(* Logix 5000 AddOnInstructionDefinition export Banner_T30RKU_Param_v4; software revision 33.00; part 2 of 3 *)
(* tags used below, declared in another part *)
   T30RKU : Banner_T30RKU_v4;
   Port_Data : Banner_IOL_Port_v4;
   Port : DINT;
   Local_Control : DINT;
   Command_Being_Processed : BOOL;
   Update_Archive : BOOL;
   Index_Write_Inprocess : DINT;
   Index_Write_Control : DINT;
   Inprocess_Index : DINT;
(* Banner_T30RKU_Param_v4, continued *)

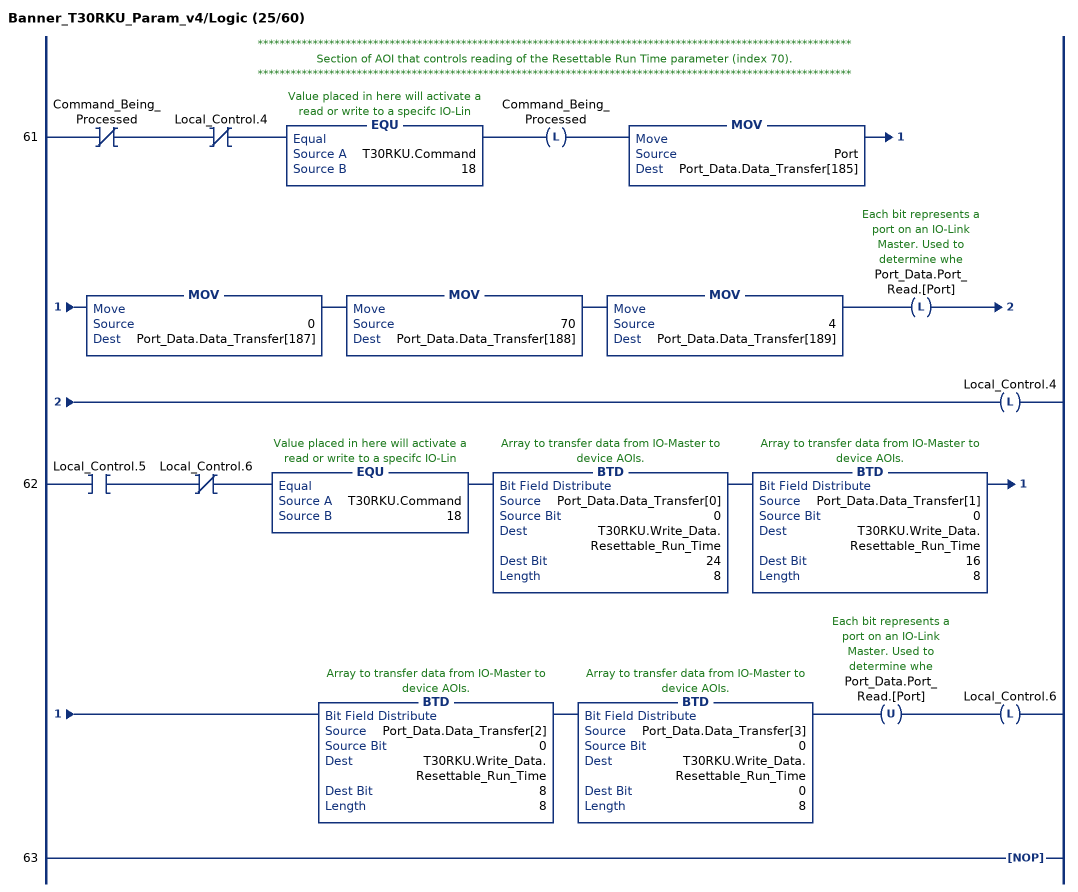
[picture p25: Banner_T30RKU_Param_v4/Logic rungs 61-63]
   // ************************************************************************************************************
   // Section of AOI that controls reading of the Resettable Run Time parameter (index 70).
   // ************************************************************************************************************
   61: XIO(Command_Being_Processed)XIO(Local_Control.4)EQU(T30RKU.Command,18)OTL(Command_Being_Processed)MOV(Port,Port_Data.Data_Transfer[185])MOV(0,Port_Data.Data_Transfer[187])MOV(70,Port_Data.Data_Transfer[188])MOV(4,Port_Data.Data_Transfer[189])OTL(Port_Data.Port_Read.[Port])OTL(Local_Control.4);
   62: XIC(Local_Control.5)XIO(Local_Control.6)EQU(T30RKU.Command,18)BTD(Port_Data.Data_Transfer[0],0,T30RKU.Write_Data.Resettable_Run_Time,24,8)BTD(Port_Data.Data_Transfer[1],0,T30RKU.Write_Data.Resettable_Run_Time,16,8)BTD(Port_Data.Data_Transfer[2],0,T30RKU.Write_Data.Resettable_Run_Time,8,8)BTD(Port_Data.Data_Transfer[3],0,T30RKU.Write_Data.Resettable_Run_Time,0,8)OTU(Port_Data.Port_Read.[Port])OTL(Local_Control.6);
   63: NOP();
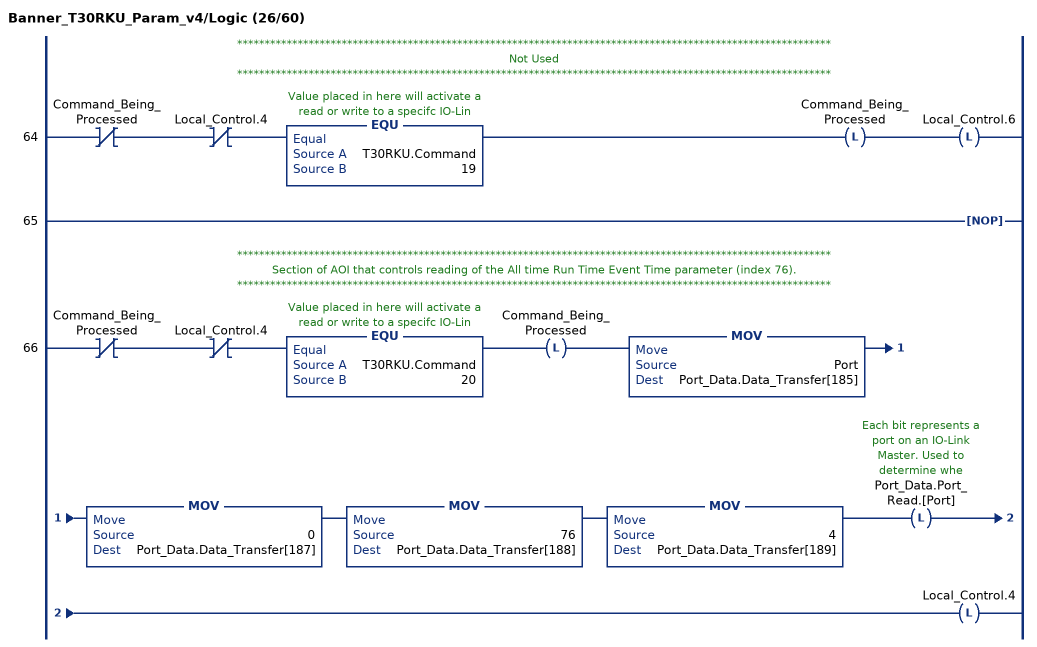
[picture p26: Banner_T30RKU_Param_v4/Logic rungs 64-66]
   // ************************************************************************************************************
   // Not Used
   // ************************************************************************************************************
   64: XIO(Command_Being_Processed)XIO(Local_Control.4)EQU(T30RKU.Command,19)OTL(Command_Being_Processed)OTL(Local_Control.6);
   65: NOP();
   // ************************************************************************************************************
   // Section of AOI that controls reading of the All time Run Time Event Time parameter (index 76).
   // ************************************************************************************************************
   66: XIO(Command_Being_Processed)XIO(Local_Control.4)EQU(T30RKU.Command,20)OTL(Command_Being_Processed)MOV(Port,Port_Data.Data_Transfer[185])MOV(0,Port_Data.Data_Transfer[187])MOV(76,Port_Data.Data_Transfer[188])MOV(4,Port_Data.Data_Transfer[189])OTL(Port_Data.Port_Read.[Port])OTL(Local_Control.4);
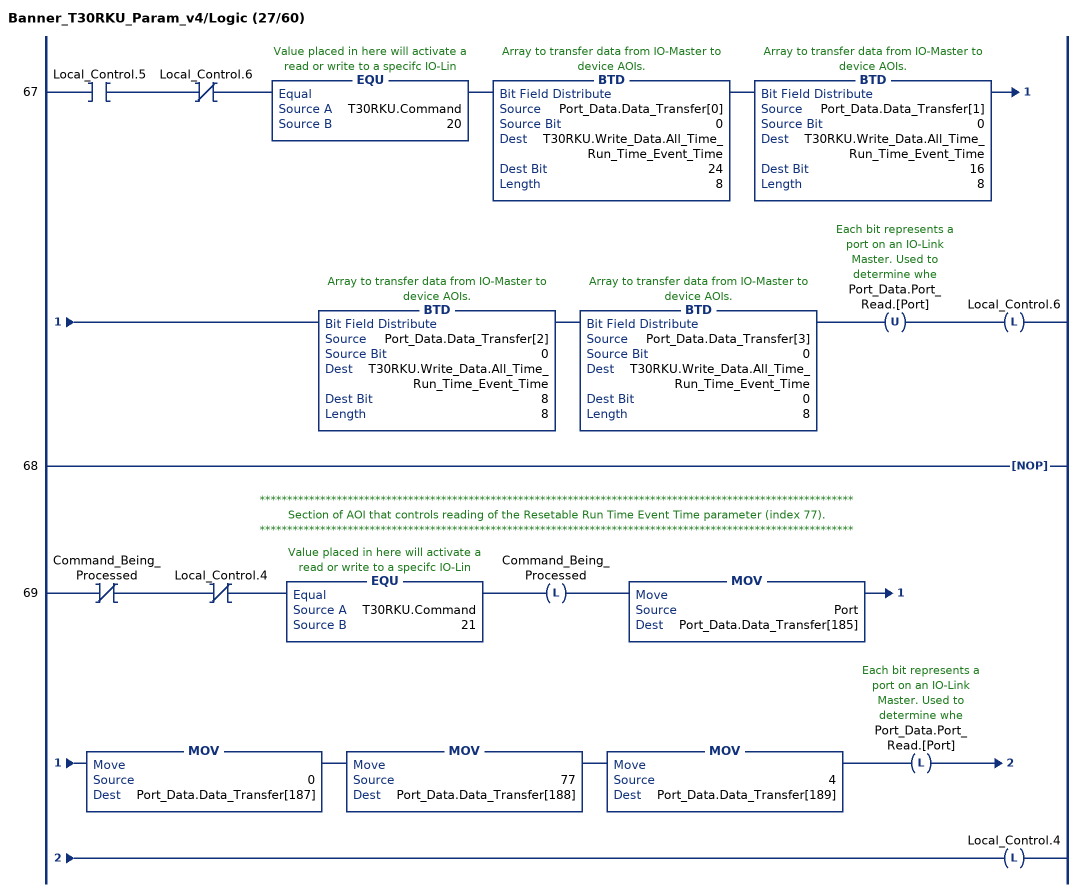
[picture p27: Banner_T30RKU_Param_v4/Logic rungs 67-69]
   67: XIC(Local_Control.5)XIO(Local_Control.6)EQU(T30RKU.Command,20)BTD(Port_Data.Data_Transfer[0],0,T30RKU.Write_Data.All_Time_Run_Time_Event_Time,24,8)BTD(Port_Data.Data_Transfer[1],0,T30RKU.Write_Data.All_Time_Run_Time_Event_Time,16,8)BTD(Port_Data.Data_Transfer[2],0,T30RKU.Write_Data.All_Time_Run_Time_Event_Time,8,8)BTD(Port_Data.Data_Transfer[3],0,T30RKU.Write_Data.All_Time_Run_Time_Event_Time,0,8)OTU(Port_Data.Port_Read.[Port])OTL(Local_Control.6);
   68: NOP();
   // ************************************************************************************************************
   // Section of AOI that controls reading of the Resetable Run Time Event Time parameter (index 77).
   // ************************************************************************************************************
   69: XIO(Command_Being_Processed)XIO(Local_Control.4)EQU(T30RKU.Command,21)OTL(Command_Being_Processed)MOV(Port,Port_Data.Data_Transfer[185])MOV(0,Port_Data.Data_Transfer[187])MOV(77,Port_Data.Data_Transfer[188])MOV(4,Port_Data.Data_Transfer[189])OTL(Port_Data.Port_Read.[Port])OTL(Local_Control.4);
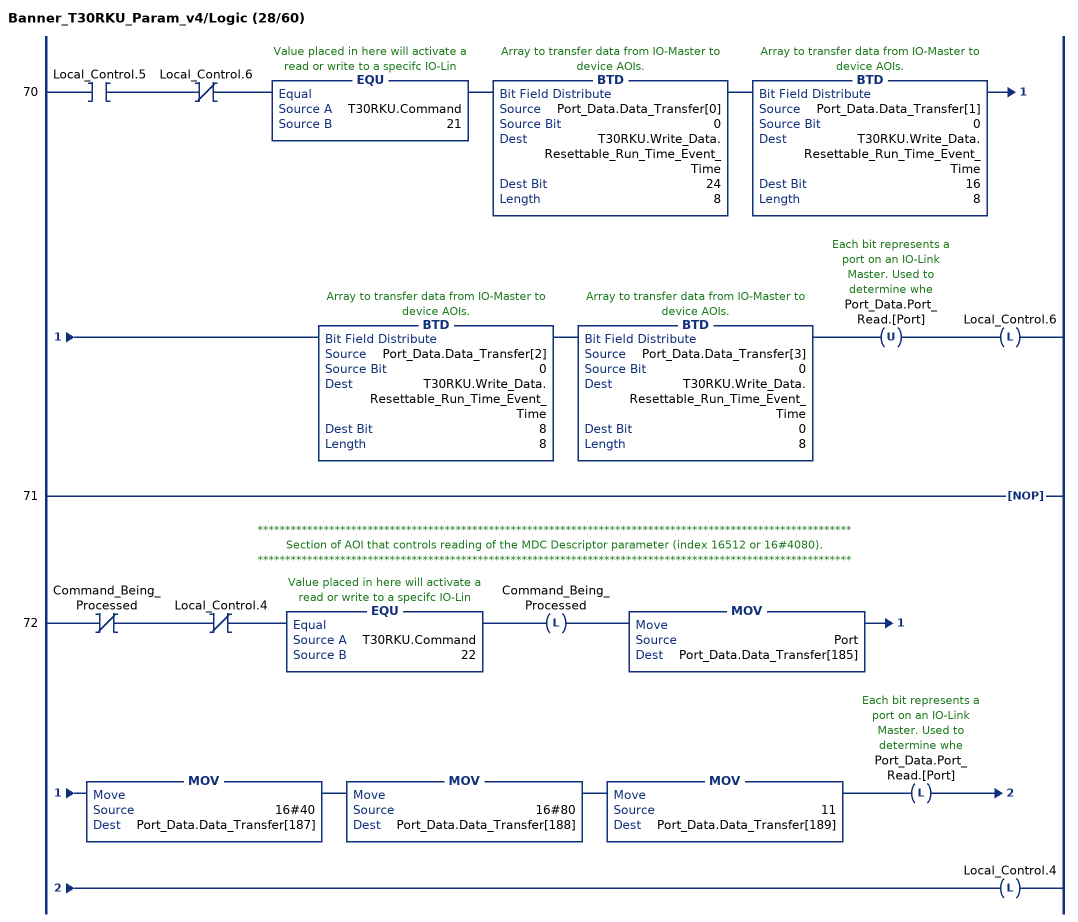
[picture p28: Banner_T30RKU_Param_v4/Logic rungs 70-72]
   70: XIC(Local_Control.5)XIO(Local_Control.6)EQU(T30RKU.Command,21)BTD(Port_Data.Data_Transfer[0],0,T30RKU.Write_Data.Resettable_Run_Time_Event_Time,24,8)BTD(Port_Data.Data_Transfer[1],0,T30RKU.Write_Data.Resettable_Run_Time_Event_Time,16,8)BTD(Port_Data.Data_Transfer[2],0,T30RKU.Write_Data.Resettable_Run_Time_Event_Time,8,8)BTD(Port_Data.Data_Transfer[3],0,T30RKU.Write_Data.Resettable_Run_Time_Event_Time,0,8)OTU(Port_Data.Port_Read.[Port])OTL(Local_Control.6);
   71: NOP();
   // ************************************************************************************************************
   // Section of AOI that controls reading of the MDC Descriptor parameter (index 16512 or 16#4080).
   // ************************************************************************************************************
   72: XIO(Command_Being_Processed)XIO(Local_Control.4)EQU(T30RKU.Command,22)OTL(Command_Being_Processed)MOV(Port,Port_Data.Data_Transfer[185])MOV(16#40,Port_Data.Data_Transfer[187])MOV(16#80,Port_Data.Data_Transfer[188])MOV(11,Port_Data.Data_Transfer[189])OTL(Port_Data.Port_Read.[Port])OTL(Local_Control.4);
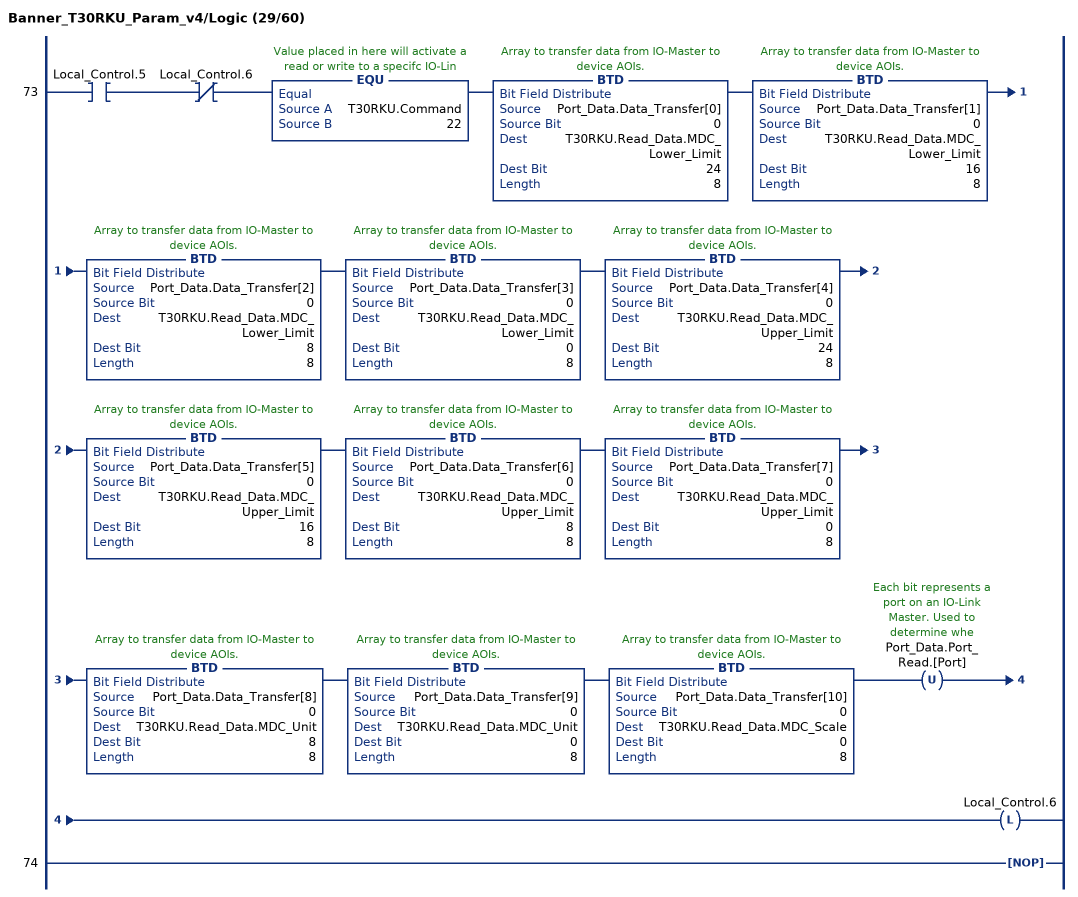
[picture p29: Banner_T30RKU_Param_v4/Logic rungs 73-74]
   73: XIC(Local_Control.5)XIO(Local_Control.6)EQU(T30RKU.Command,22)BTD(Port_Data.Data_Transfer[0],0,T30RKU.Read_Data.MDC_Lower_Limit,24,8)BTD(Port_Data.Data_Transfer[1],0,T30RKU.Read_Data.MDC_Lower_Limit,16,8)BTD(Port_Data.Data_Transfer[2],0,T30RKU.Read_Data.MDC_Lower_Limit,8,8)BTD(Port_Data.Data_Transfer[3],0,T30RKU.Read_Data.MDC_Lower_Limit,0,8)BTD(Port_Data.Data_Transfer[4],0,T30RKU.Read_Data.MDC_Upper_Limit,24,8)BTD(Port_Data.Data_Transfer[5],0,T30RKU.Read_Data.MDC_Upper_Limit,16,8)BTD(Port_Data.Data_Transfer[6],0,T30RKU.Read_Data.MDC_Upper_Limit,8,8)BTD(Port_Data.Data_Transfer[7],0,T30RKU.Read_Data.MDC_Upper_Limit,0,8)BTD(Port_Data.Data_Transfer[8],0,T30RKU.Read_Data.MDC_Unit,8,8)BTD(Port_Data.Data_Transfer[9],0,T30RKU.Read_Data.MDC_Unit,0,8)BTD(Port_Data.Data_Transfer[10],0,T30RKU.Read_Data.MDC_Scale,0,8)OTU(Port_Data.Port_Read.[Port])OTL(Local_Control.6);
   74: NOP();
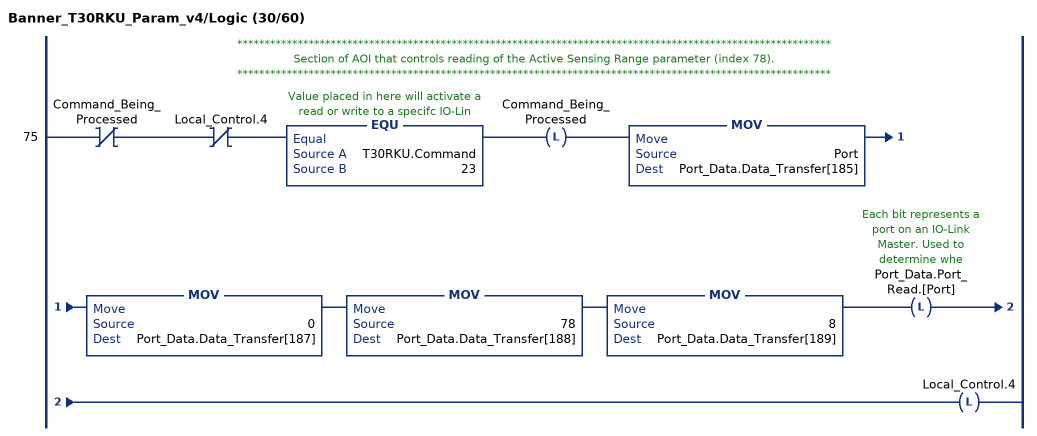
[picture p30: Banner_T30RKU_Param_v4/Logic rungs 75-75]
   // ************************************************************************************************************
   // Section of AOI that controls reading of the Active Sensing Range parameter (index 78).
   // ************************************************************************************************************
   75: XIO(Command_Being_Processed)XIO(Local_Control.4)EQU(T30RKU.Command,23)OTL(Command_Being_Processed)MOV(Port,Port_Data.Data_Transfer[185])MOV(0,Port_Data.Data_Transfer[187])MOV(78,Port_Data.Data_Transfer[188])MOV(8,Port_Data.Data_Transfer[189])OTL(Port_Data.Port_Read.[Port])OTL(Local_Control.4);
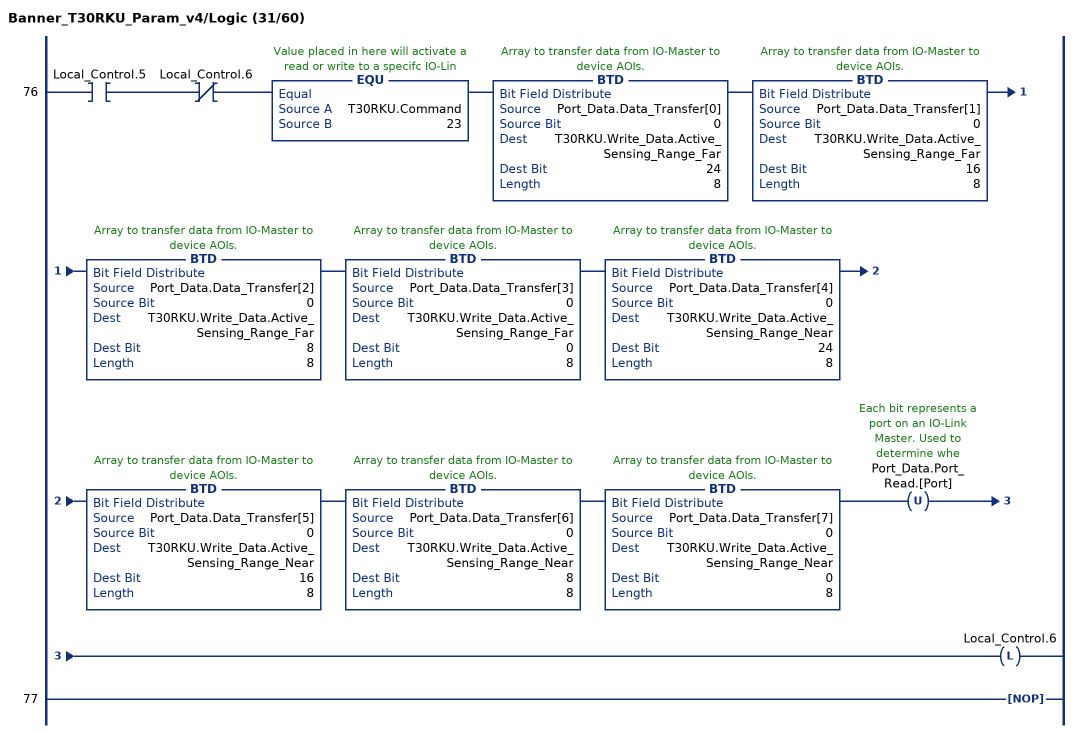
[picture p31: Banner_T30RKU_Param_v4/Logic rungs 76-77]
   76: XIC(Local_Control.5)XIO(Local_Control.6)EQU(T30RKU.Command,23)BTD(Port_Data.Data_Transfer[0],0,T30RKU.Write_Data.Active_Sensing_Range_Far,24,8)BTD(Port_Data.Data_Transfer[1],0,T30RKU.Write_Data.Active_Sensing_Range_Far,16,8)BTD(Port_Data.Data_Transfer[2],0,T30RKU.Write_Data.Active_Sensing_Range_Far,8,8)BTD(Port_Data.Data_Transfer[3],0,T30RKU.Write_Data.Active_Sensing_Range_Far,0,8)BTD(Port_Data.Data_Transfer[4],0,T30RKU.Write_Data.Active_Sensing_Range_Near,24,8)BTD(Port_Data.Data_Transfer[5],0,T30RKU.Write_Data.Active_Sensing_Range_Near,16,8)BTD(Port_Data.Data_Transfer[6],0,T30RKU.Write_Data.Active_Sensing_Range_Near,8,8)BTD(Port_Data.Data_Transfer[7],0,T30RKU.Write_Data.Active_Sensing_Range_Near,0,8)OTU(Port_Data.Port_Read.[Port])OTL(Local_Control.6);
   77: NOP();
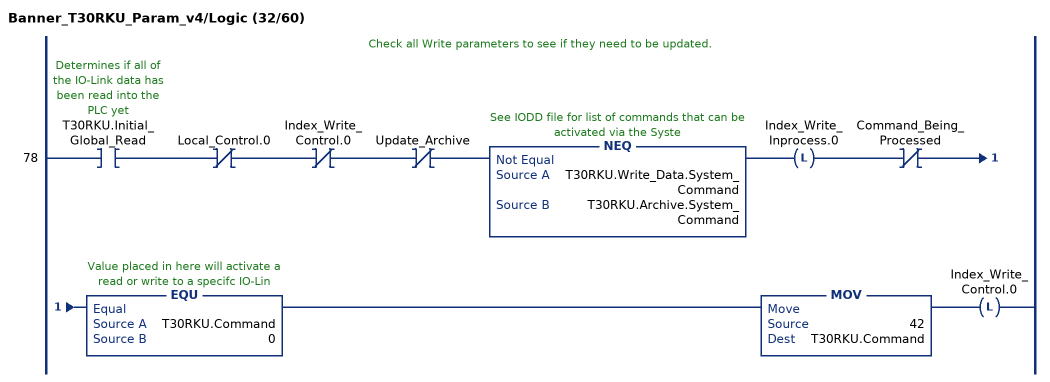
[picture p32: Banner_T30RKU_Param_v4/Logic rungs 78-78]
   // Check all Write parameters to see if they need to be updated.
   78: XIC(T30RKU.Initial_Global_Read)XIO(Local_Control.0)XIO(Index_Write_Control.0)XIO(Update_Archive)NEQ(T30RKU.Write_Data.System_Command,T30RKU.Archive.System_Command)OTL(Index_Write_Inprocess.0)XIO(Command_Being_Processed)EQU(T30RKU.Command,0)MOV(42,T30RKU.Command)OTL(Index_Write_Control.0);
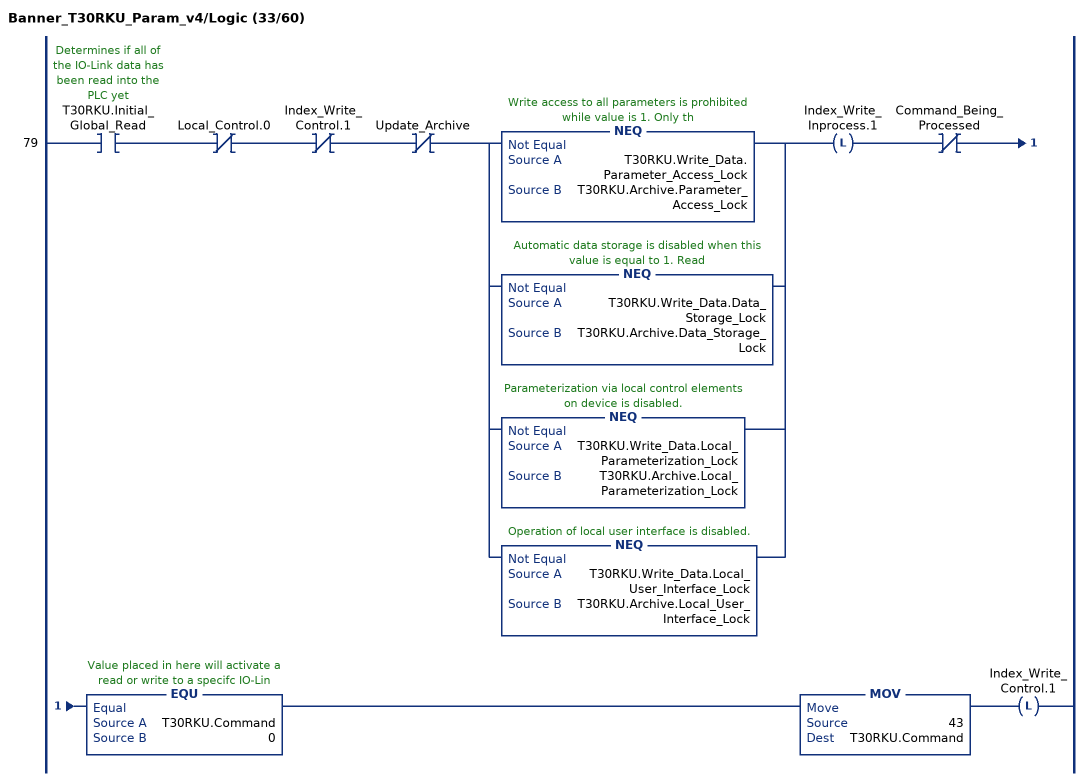
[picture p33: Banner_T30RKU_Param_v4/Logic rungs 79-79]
   79: XIC(T30RKU.Initial_Global_Read)XIO(Local_Control.0)XIO(Index_Write_Control.1)XIO(Update_Archive)[NEQ(T30RKU.Write_Data.Parameter_Access_Lock,T30RKU.Archive.Parameter_Access_Lock) ,NEQ(T30RKU.Write_Data.Data_Storage_Lock,T30RKU.Archive.Data_Storage_Lock) ,NEQ(T30RKU.Write_Data.Local_Parameterization_Lock,T30RKU.Archive.Local_Parameterization_Lock) ,NEQ(T30RKU.Write_Data.Local_User_Interface_Lock,T30RKU.Archive.Local_User_Interface_Lock) ]OTL(Index_Write_Inprocess.1)XIO(Command_Being_Processed)EQU(T30RKU.Command,0)MOV(43,T30RKU.Command)OTL(Index_Write_Control.1);
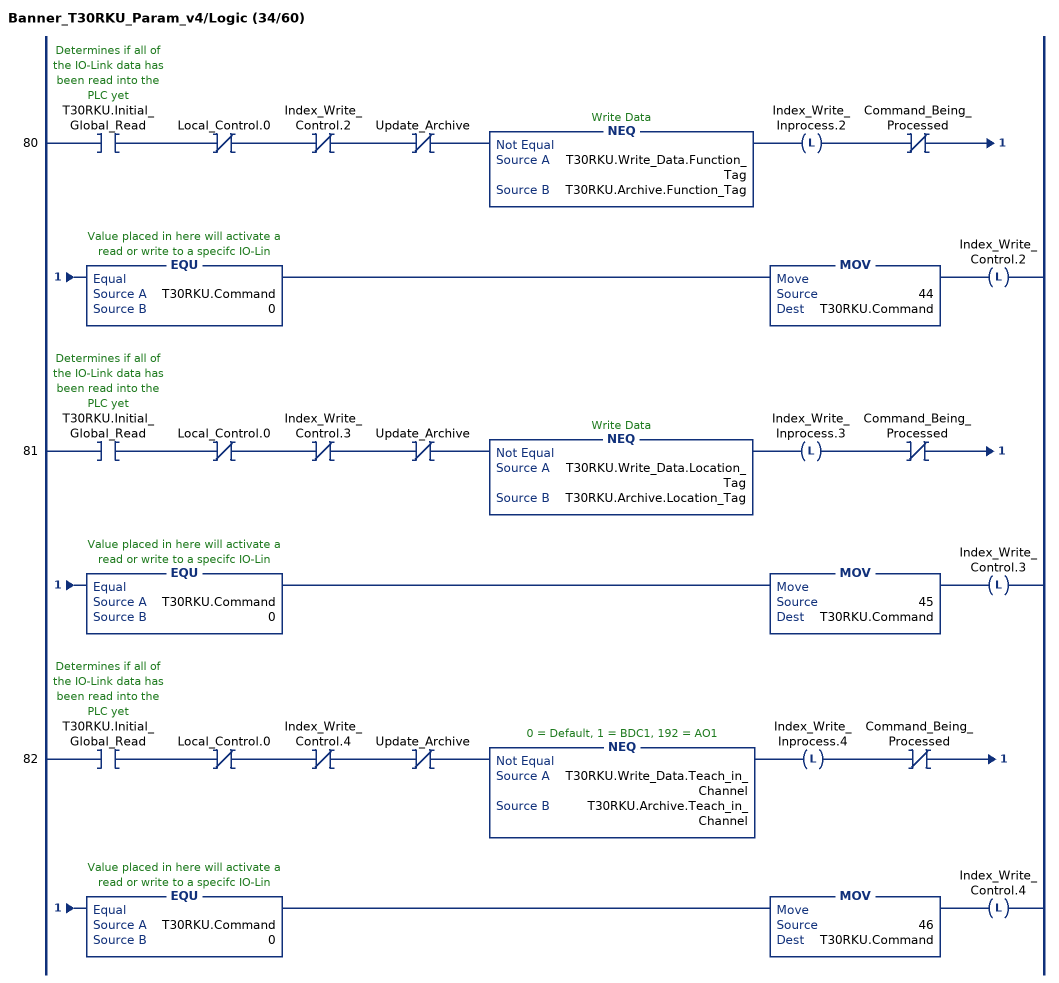
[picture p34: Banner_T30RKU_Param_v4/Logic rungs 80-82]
   80: XIC(T30RKU.Initial_Global_Read)XIO(Local_Control.0)XIO(Index_Write_Control.2)XIO(Update_Archive)NEQ(T30RKU.Write_Data.Function_Tag,T30RKU.Archive.Function_Tag)OTL(Index_Write_Inprocess.2)XIO(Command_Being_Processed)EQU(T30RKU.Command,0)MOV(44,T30RKU.Command)OTL(Index_Write_Control.2);
   81: XIC(T30RKU.Initial_Global_Read)XIO(Local_Control.0)XIO(Index_Write_Control.3)XIO(Update_Archive)NEQ(T30RKU.Write_Data.Location_Tag,T30RKU.Archive.Location_Tag)OTL(Index_Write_Inprocess.3)XIO(Command_Being_Processed)EQU(T30RKU.Command,0)MOV(45,T30RKU.Command)OTL(Index_Write_Control.3);
   82: XIC(T30RKU.Initial_Global_Read)XIO(Local_Control.0)XIO(Index_Write_Control.4)XIO(Update_Archive)NEQ(T30RKU.Write_Data.Teach_in_Channel,T30RKU.Archive.Teach_in_Channel)OTL(Index_Write_Inprocess.4)XIO(Command_Being_Processed)EQU(T30RKU.Command,0)MOV(46,T30RKU.Command)OTL(Index_Write_Control.4);
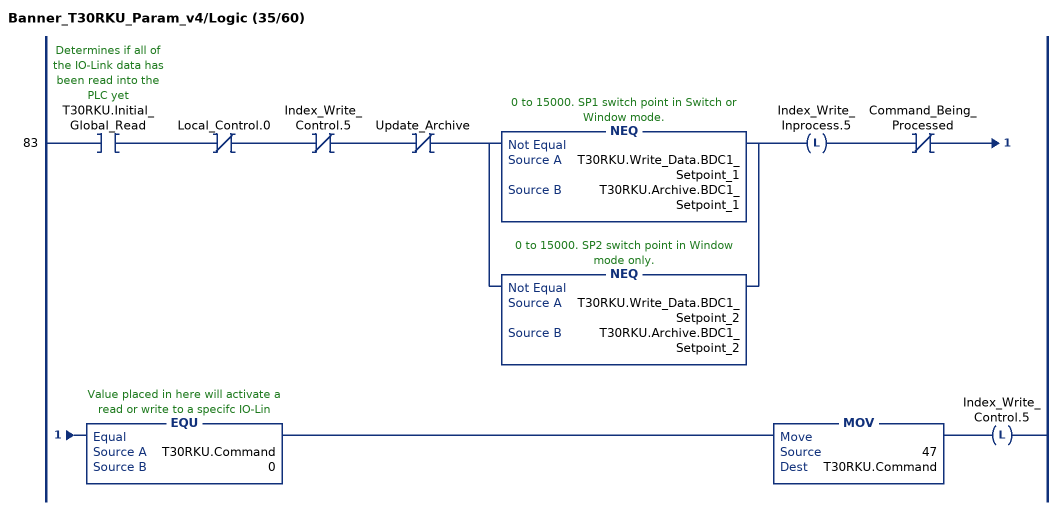
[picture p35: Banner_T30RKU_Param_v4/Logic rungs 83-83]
   83: XIC(T30RKU.Initial_Global_Read)XIO(Local_Control.0)XIO(Index_Write_Control.5)XIO(Update_Archive)[NEQ(T30RKU.Write_Data.BDC1_Setpoint_1,T30RKU.Archive.BDC1_Setpoint_1) ,NEQ(T30RKU.Write_Data.BDC1_Setpoint_2,T30RKU.Archive.BDC1_Setpoint_2) ]OTL(Index_Write_Inprocess.5)XIO(Command_Being_Processed)EQU(T30RKU.Command,0)MOV(47,T30RKU.Command)OTL(Index_Write_Control.5);
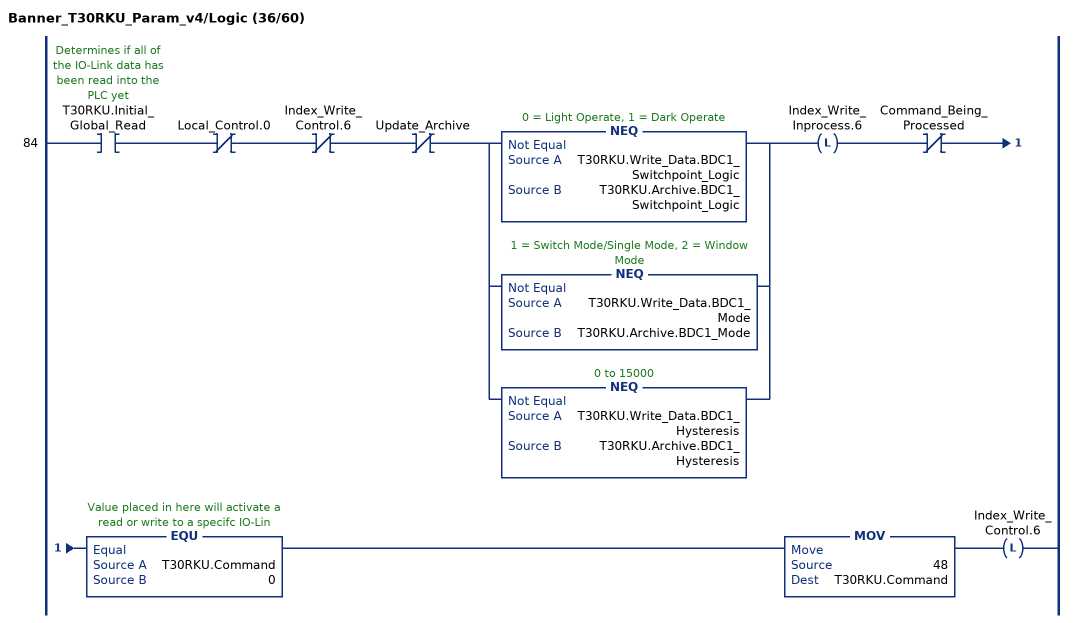
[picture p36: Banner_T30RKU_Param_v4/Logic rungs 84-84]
   84: XIC(T30RKU.Initial_Global_Read)XIO(Local_Control.0)XIO(Index_Write_Control.6)XIO(Update_Archive)[NEQ(T30RKU.Write_Data.BDC1_Switchpoint_Logic,T30RKU.Archive.BDC1_Switchpoint_Logic) ,NEQ(T30RKU.Write_Data.BDC1_Mode,T30RKU.Archive.BDC1_Mode) ,NEQ(T30RKU.Write_Data.BDC1_Hysteresis,T30RKU.Archive.BDC1_Hysteresis) ]OTL(Index_Write_Inprocess.6)XIO(Command_Being_Processed)EQU(T30RKU.Command,0)MOV(48,T30RKU.Command)OTL(Index_Write_Control.6);
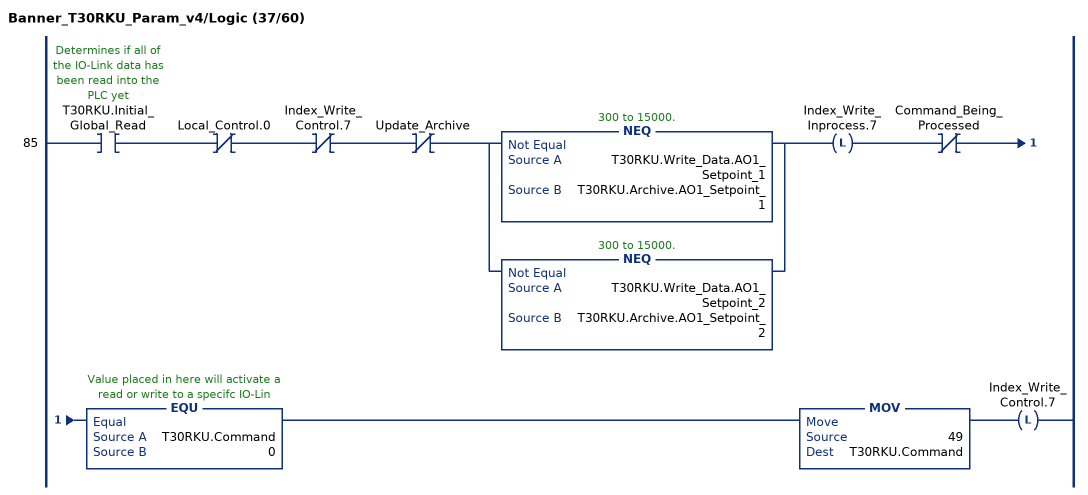
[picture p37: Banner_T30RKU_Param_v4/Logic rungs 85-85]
   85: XIC(T30RKU.Initial_Global_Read)XIO(Local_Control.0)XIO(Index_Write_Control.7)XIO(Update_Archive)[NEQ(T30RKU.Write_Data.AO1_Setpoint_1,T30RKU.Archive.AO1_Setpoint_1) ,NEQ(T30RKU.Write_Data.AO1_Setpoint_2,T30RKU.Archive.AO1_Setpoint_2) ]OTL(Index_Write_Inprocess.7)XIO(Command_Being_Processed)EQU(T30RKU.Command,0)MOV(49,T30RKU.Command)OTL(Index_Write_Control.7);
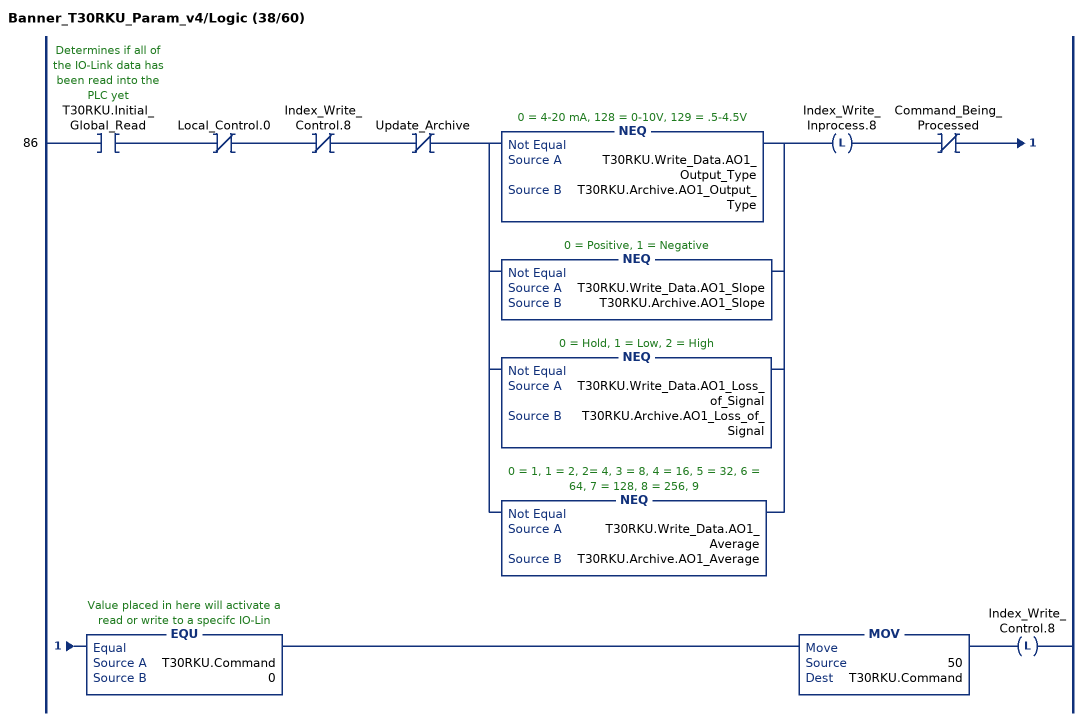
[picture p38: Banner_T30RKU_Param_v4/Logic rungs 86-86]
   86: XIC(T30RKU.Initial_Global_Read)XIO(Local_Control.0)XIO(Index_Write_Control.8)XIO(Update_Archive)[NEQ(T30RKU.Write_Data.AO1_Output_Type,T30RKU.Archive.AO1_Output_Type) ,NEQ(T30RKU.Write_Data.AO1_Slope,T30RKU.Archive.AO1_Slope) ,NEQ(T30RKU.Write_Data.AO1_Loss_of_Signal,T30RKU.Archive.AO1_Loss_of_Signal) ,NEQ(T30RKU.Write_Data.AO1_Average,T30RKU.Archive.AO1_Average) ]OTL(Index_Write_Inprocess.8)XIO(Command_Being_Processed)EQU(T30RKU.Command,0)MOV(50,T30RKU.Command)OTL(Index_Write_Control.8);
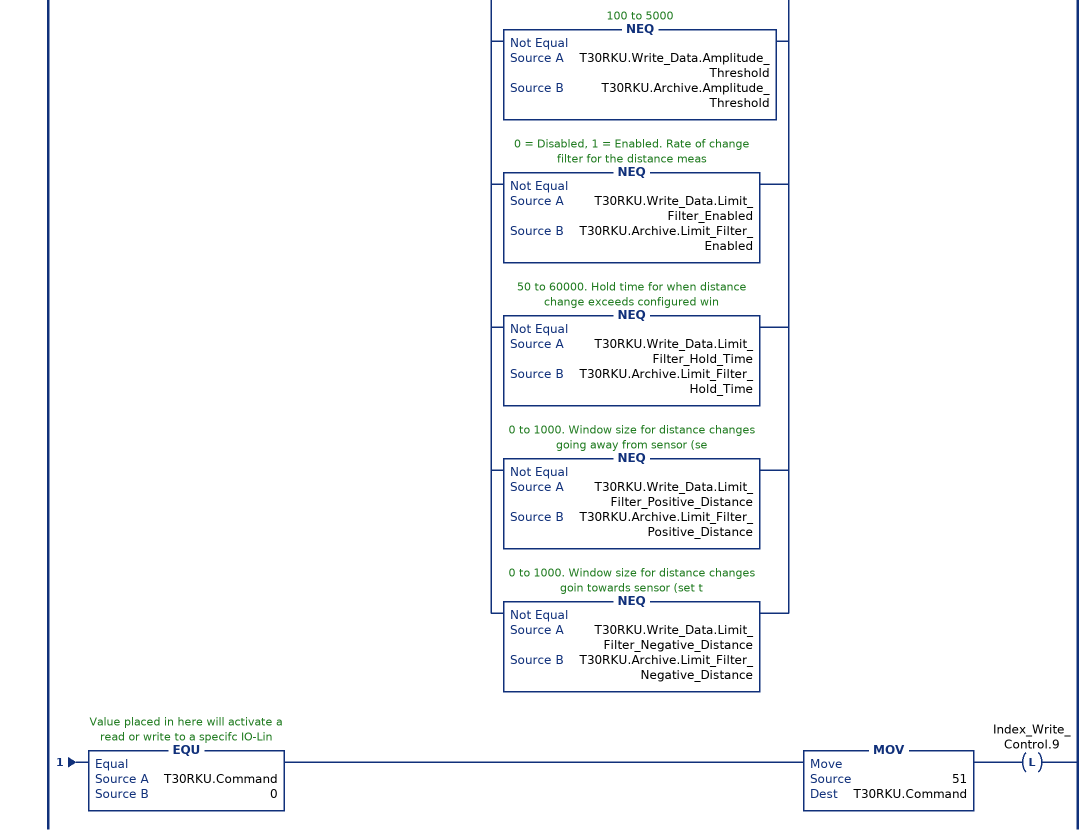
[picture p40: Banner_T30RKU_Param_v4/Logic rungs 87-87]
   87: XIC(T30RKU.Initial_Global_Read)XIO(Local_Control.0)XIO(Index_Write_Control.9)XIO(Update_Archive)[NEQ(T30RKU.Write_Data.Response_Speed,T30RKU.Archive.Response_Speed) ,NEQ(T30RKU.Write_Data.Peak_Select_Mode,T30RKU.Archive.Peak_Select_Mode) ,NEQ(T30RKU.Write_Data.Sensor_Lockout,T30RKU.Archive.Sensor_Lockout) ,NEQ(T30RKU.Write_Data.Output_Polarity,T30RKU.Archive.Output_Polarity) ,NEQ(T30RKU.Write_Data.Process_Data_Filter_Time,T30RKU.Archive.Process_Data_Filter_Time) ,NEQ(T30RKU.Write_Data.Process_Data_Layout,T30RKU.Archive.Process_Data_Layout) ,NEQ(T30RKU.Write_Data.Remote_Input_Mode,T30RKU.Archive.Remote_Input_Mode) ,NEQ(T30RKU.Write_Data.Amplitude_Threshold,T30RKU.Archive.Amplitude_Threshold) ,NEQ(T30RKU.Write_Data.Limit_Filter_Enabled,T30RKU.Archive.Limit_Filter_Enabled) ,NEQ(T30RKU.Write_Data.Limit_Filter_Hold_Time,T30RKU.Archive.Limit_Filter_Hold_Time) ,NEQ(T30RKU.Write_Data.Limit_Filter_Positive_Distance,T30RKU.Archive.Limit_Filter_Positive_Distance) ,NEQ(T30RKU.Write_Data.Limit_Filter_Negative_Distance,T30RKU.Archive.Limit_Filter_Negative_Distance) ]OTL(Index_Write_Inprocess.9)XIO(Command_Being_Processed)EQU(T30RKU.Command,0)MOV(51,T30RKU.Command)OTL(Index_Write_Control.9);
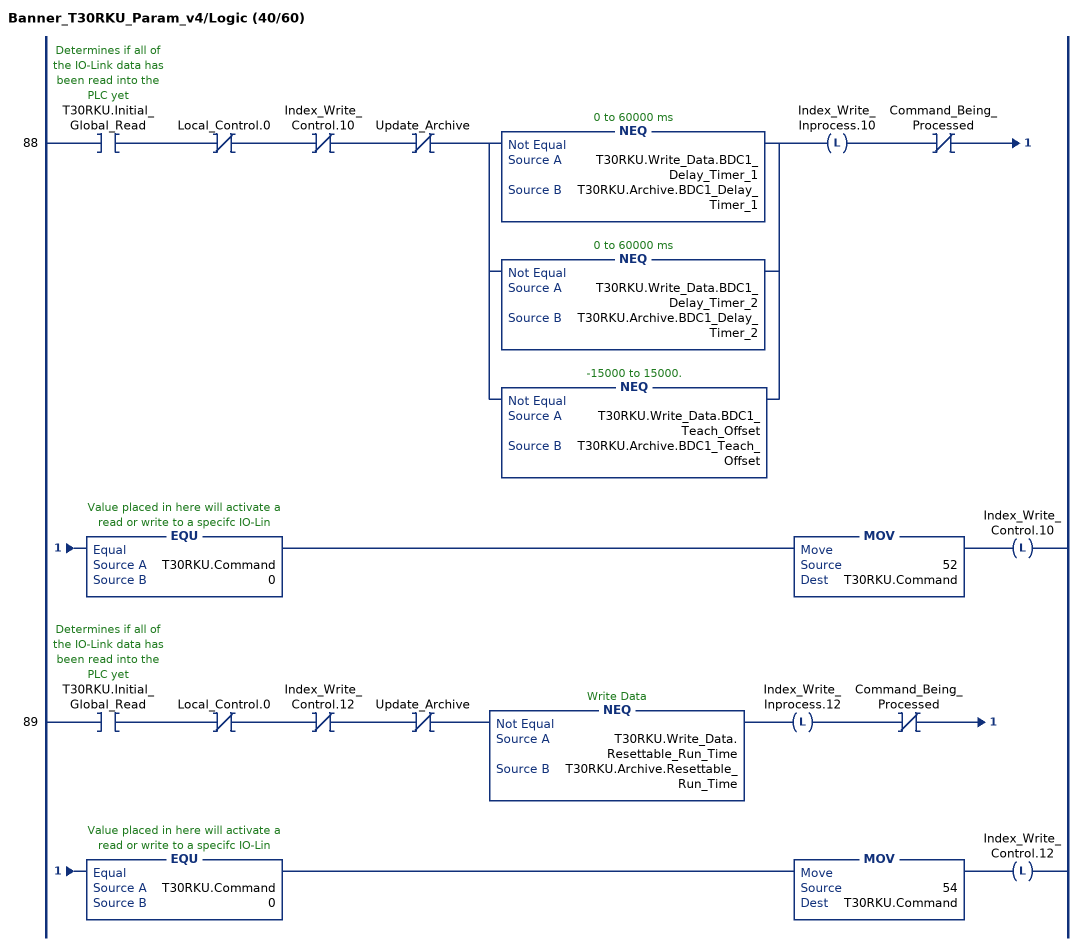
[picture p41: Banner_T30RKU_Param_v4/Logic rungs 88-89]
   88: XIC(T30RKU.Initial_Global_Read)XIO(Local_Control.0)XIO(Index_Write_Control.10)XIO(Update_Archive)[NEQ(T30RKU.Write_Data.BDC1_Delay_Timer_1,T30RKU.Archive.BDC1_Delay_Timer_1) ,NEQ(T30RKU.Write_Data.BDC1_Delay_Timer_2,T30RKU.Archive.BDC1_Delay_Timer_2) ,NEQ(T30RKU.Write_Data.BDC1_Teach_Offset,T30RKU.Archive.BDC1_Teach_Offset) ]OTL(Index_Write_Inprocess.10)XIO(Command_Being_Processed)EQU(T30RKU.Command,0)MOV(52,T30RKU.Command)OTL(Index_Write_Control.10);
   89: XIC(T30RKU.Initial_Global_Read)XIO(Local_Control.0)XIO(Index_Write_Control.12)XIO(Update_Archive)NEQ(T30RKU.Write_Data.Resettable_Run_Time,T30RKU.Archive.Resettable_Run_Time)OTL(Index_Write_Inprocess.12)XIO(Command_Being_Processed)EQU(T30RKU.Command,0)MOV(54,T30RKU.Command)OTL(Index_Write_Control.12);
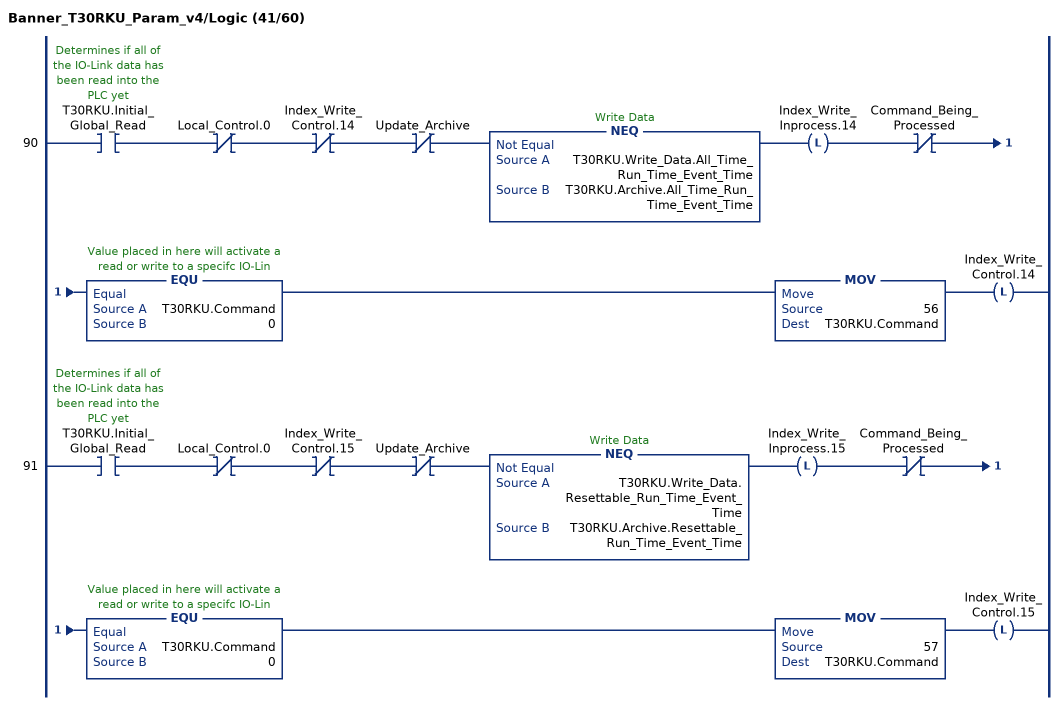
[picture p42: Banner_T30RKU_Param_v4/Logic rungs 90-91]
   90: XIC(T30RKU.Initial_Global_Read)XIO(Local_Control.0)XIO(Index_Write_Control.14)XIO(Update_Archive)NEQ(T30RKU.Write_Data.All_Time_Run_Time_Event_Time,T30RKU.Archive.All_Time_Run_Time_Event_Time)OTL(Index_Write_Inprocess.14)XIO(Command_Being_Processed)EQU(T30RKU.Command,0)MOV(56,T30RKU.Command)OTL(Index_Write_Control.14);
   91: XIC(T30RKU.Initial_Global_Read)XIO(Local_Control.0)XIO(Index_Write_Control.15)XIO(Update_Archive)NEQ(T30RKU.Write_Data.Resettable_Run_Time_Event_Time,T30RKU.Archive.Resettable_Run_Time_Event_Time)OTL(Index_Write_Inprocess.15)XIO(Command_Being_Processed)EQU(T30RKU.Command,0)MOV(57,T30RKU.Command)OTL(Index_Write_Control.15);
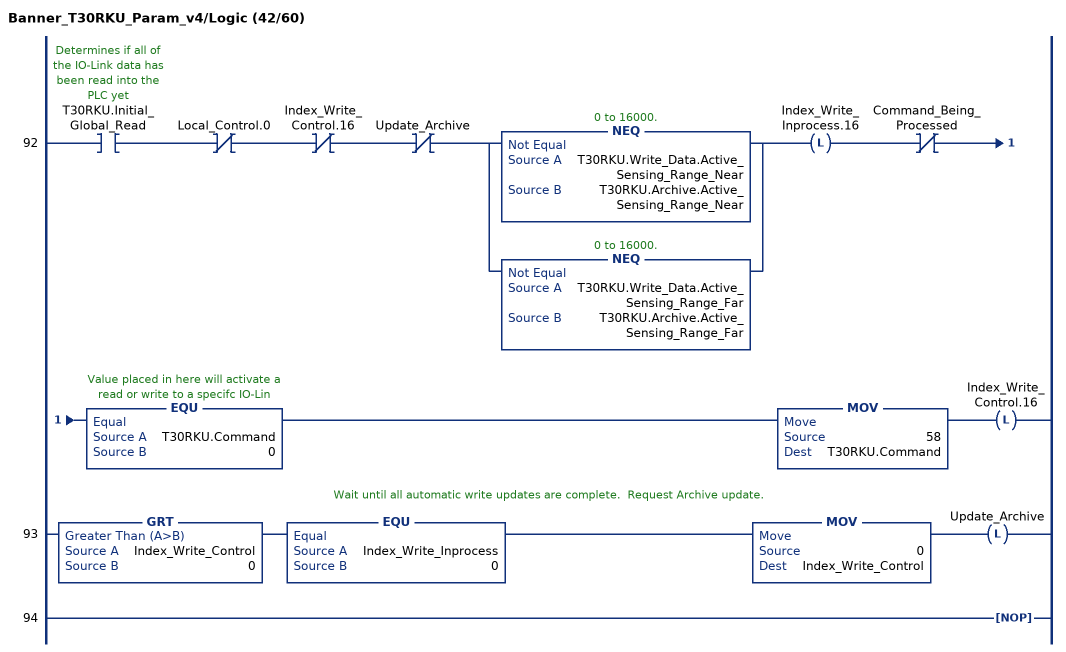
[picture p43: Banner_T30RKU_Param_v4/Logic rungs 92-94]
   92: XIC(T30RKU.Initial_Global_Read)XIO(Local_Control.0)XIO(Index_Write_Control.16)XIO(Update_Archive)[NEQ(T30RKU.Write_Data.Active_Sensing_Range_Near,T30RKU.Archive.Active_Sensing_Range_Near) ,NEQ(T30RKU.Write_Data.Active_Sensing_Range_Far,T30RKU.Archive.Active_Sensing_Range_Far) ]OTL(Index_Write_Inprocess.16)XIO(Command_Being_Processed)EQU(T30RKU.Command,0)MOV(58,T30RKU.Command)OTL(Index_Write_Control.16);
   // Wait until all automatic write updates are complete.  Request Archive update.
   93: GRT(Index_Write_Control,0)EQU(Index_Write_Inprocess,0)MOV(0,Index_Write_Control)OTL(Update_Archive);
   94: NOP();
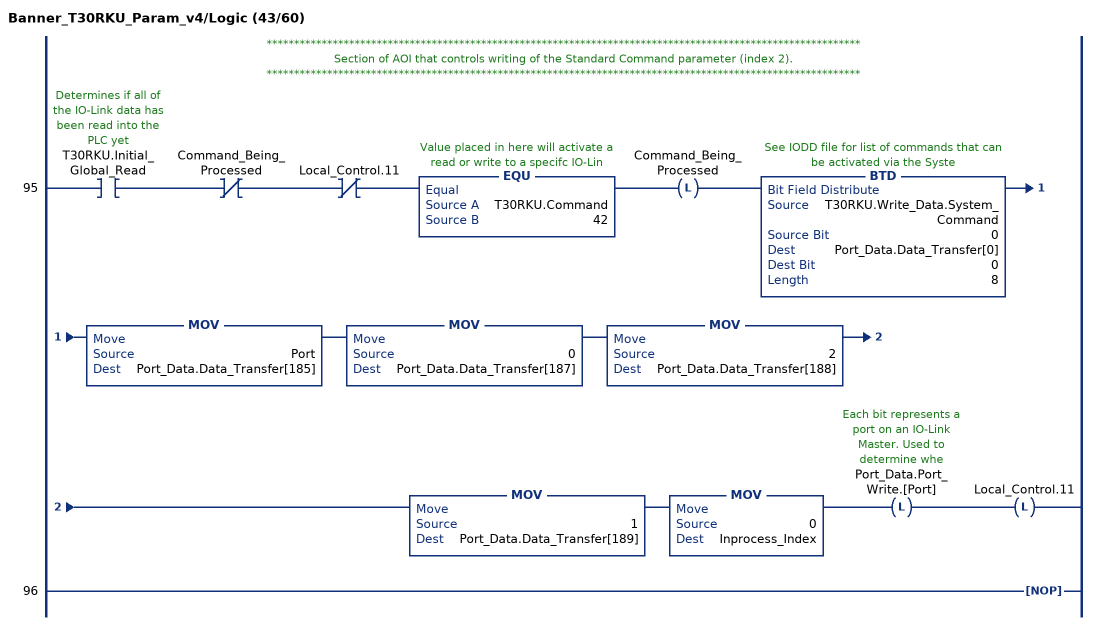
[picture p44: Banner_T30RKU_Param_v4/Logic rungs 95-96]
   // ************************************************************************************************************
   // Section of AOI that controls writing of the Standard Command parameter (index 2).
   // ************************************************************************************************************
   95: XIC(T30RKU.Initial_Global_Read)XIO(Command_Being_Processed)XIO(Local_Control.11)EQU(T30RKU.Command,42)OTL(Command_Being_Processed)BTD(T30RKU.Write_Data.System_Command,0,Port_Data.Data_Transfer[0],0,8)MOV(Port,Port_Data.Data_Transfer[185])MOV(0,Port_Data.Data_Transfer[187])MOV(2,Port_Data.Data_Transfer[188])MOV(1,Port_Data.Data_Transfer[189])MOV(0,Inprocess_Index)OTL(Port_Data.Port_Write.[Port])OTL(Local_Control.11);
   96: NOP();
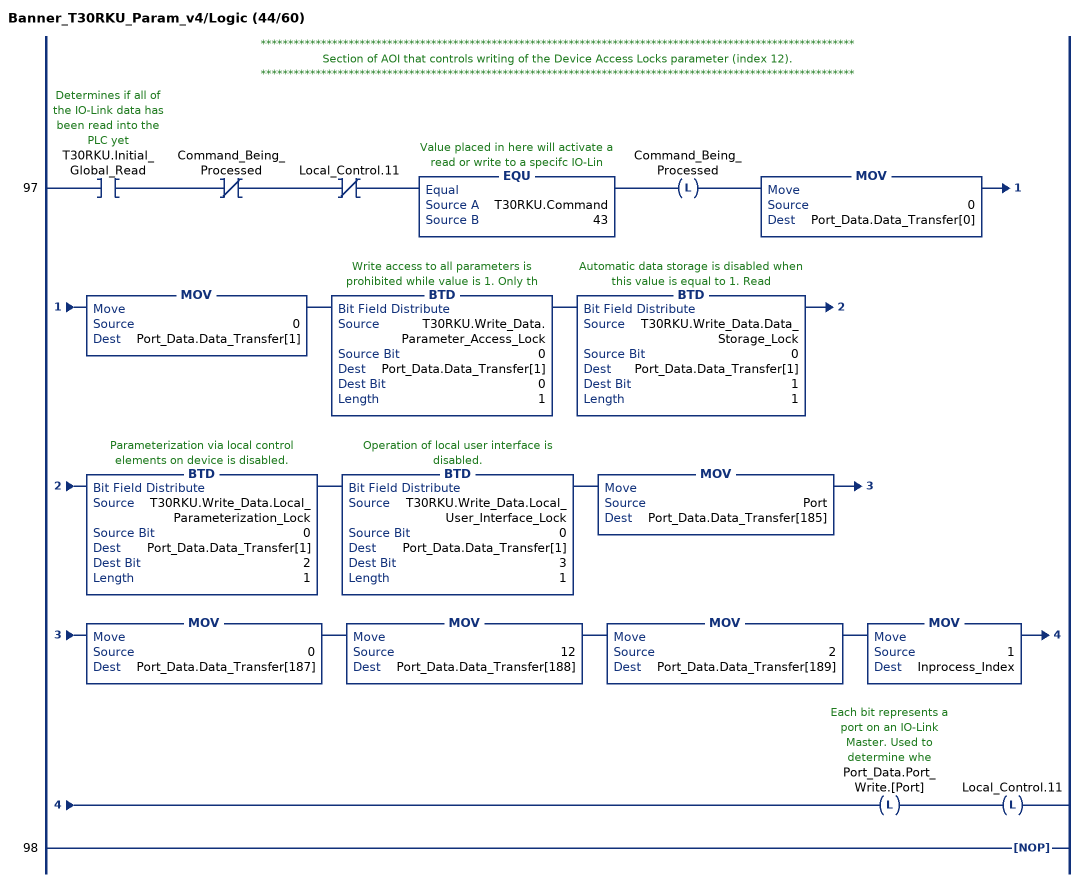
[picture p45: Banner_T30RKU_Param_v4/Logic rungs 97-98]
   // ************************************************************************************************************
   // Section of AOI that controls writing of the Device Access Locks parameter (index 12).
   // ************************************************************************************************************
   97: XIC(T30RKU.Initial_Global_Read)XIO(Command_Being_Processed)XIO(Local_Control.11)EQU(T30RKU.Command,43)OTL(Command_Being_Processed)MOV(0,Port_Data.Data_Transfer[0])MOV(0,Port_Data.Data_Transfer[1])BTD(T30RKU.Write_Data.Parameter_Access_Lock,0,Port_Data.Data_Transfer[1],0,1)BTD(T30RKU.Write_Data.Data_Storage_Lock,0,Port_Data.Data_Transfer[1],1,1)BTD(T30RKU.Write_Data.Local_Parameterization_Lock,0,Port_Data.Data_Transfer[1],2,1)BTD(T30RKU.Write_Data.Local_User_Interface_Lock,0,Port_Data.Data_Transfer[1],3,1)MOV(Port,Port_Data.Data_Transfer[185])MOV(0,Port_Data.Data_Transfer[187])MOV(12,Port_Data.Data_Transfer[188])MOV(2,Port_Data.Data_Transfer[189])MOV(1,Inprocess_Index)OTL(Port_Data.Port_Write.[Port])OTL(Local_Control.11);
   98: NOP();
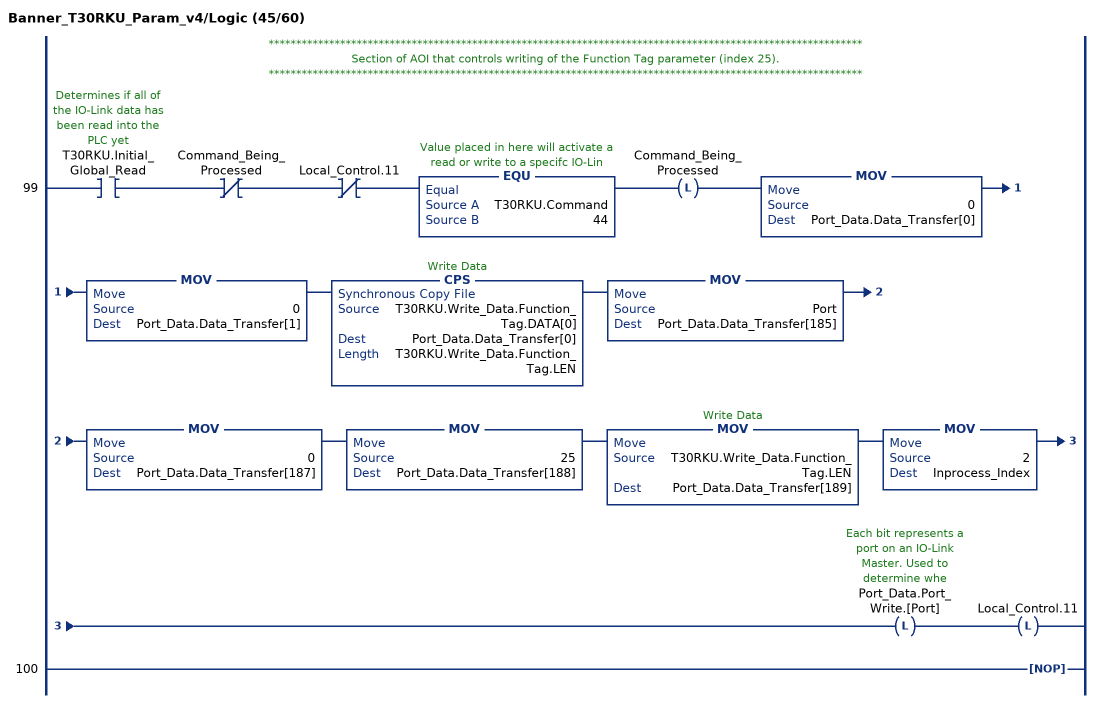
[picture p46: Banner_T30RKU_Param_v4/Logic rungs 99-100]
   // ************************************************************************************************************
   // Section of AOI that controls writing of the Function Tag parameter (index 25).
   // ************************************************************************************************************
   99: XIC(T30RKU.Initial_Global_Read)XIO(Command_Being_Processed)XIO(Local_Control.11)EQU(T30RKU.Command,44)OTL(Command_Being_Processed)MOV(0,Port_Data.Data_Transfer[0])MOV(0,Port_Data.Data_Transfer[1])CPS(T30RKU.Write_Data.Function_Tag.DATA[0],Port_Data.Data_Transfer[0],T30RKU.Write_Data.Function_Tag.LEN)MOV(Port,Port_Data.Data_Transfer[185])MOV(0,Port_Data.Data_Transfer[187])MOV(25,Port_Data.Data_Transfer[188])MOV(T30RKU.Write_Data.Function_Tag.LEN,Port_Data.Data_Transfer[189])MOV(2,Inprocess_Index)OTL(Port_Data.Port_Write.[Port])OTL(Local_Control.11);
   100: NOP();
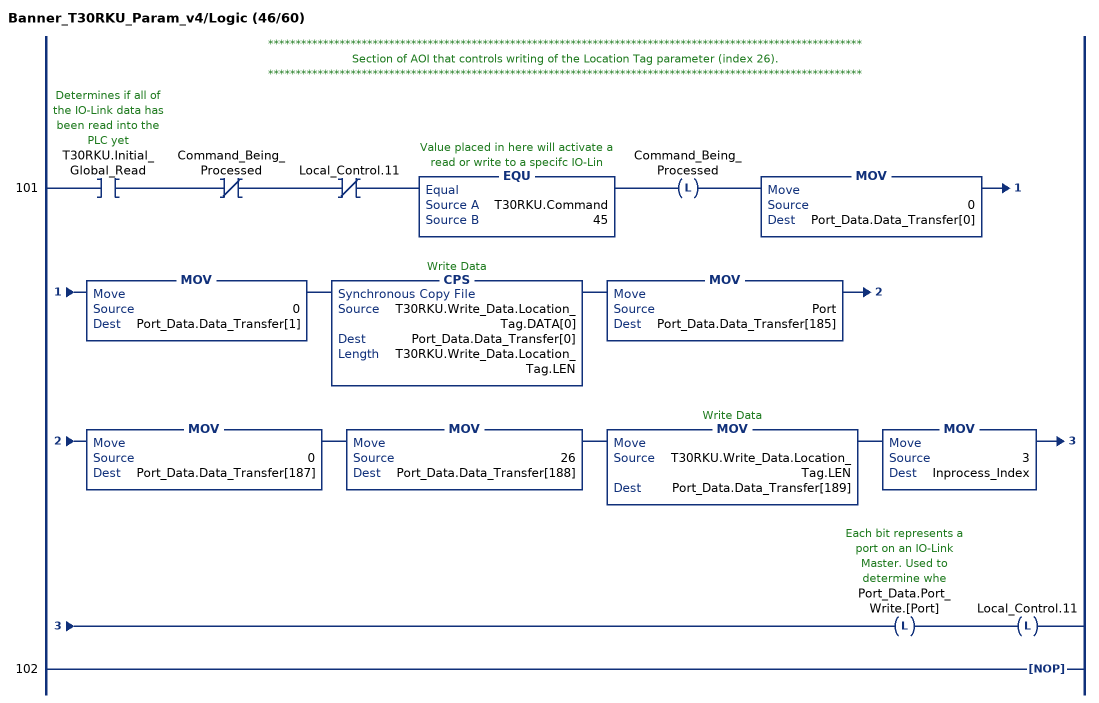
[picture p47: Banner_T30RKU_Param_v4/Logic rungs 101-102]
   // ************************************************************************************************************
   // Section of AOI that controls writing of the Location Tag parameter (index 26).
   // ************************************************************************************************************
   101: XIC(T30RKU.Initial_Global_Read)XIO(Command_Being_Processed)XIO(Local_Control.11)EQU(T30RKU.Command,45)OTL(Command_Being_Processed)MOV(0,Port_Data.Data_Transfer[0])MOV(0,Port_Data.Data_Transfer[1])CPS(T30RKU.Write_Data.Location_Tag.DATA[0],Port_Data.Data_Transfer[0],T30RKU.Write_Data.Location_Tag.LEN)MOV(Port,Port_Data.Data_Transfer[185])MOV(0,Port_Data.Data_Transfer[187])MOV(26,Port_Data.Data_Transfer[188])MOV(T30RKU.Write_Data.Location_Tag.LEN,Port_Data.Data_Transfer[189])MOV(3,Inprocess_Index)OTL(Port_Data.Port_Write.[Port])OTL(Local_Control.11);
   102: NOP();
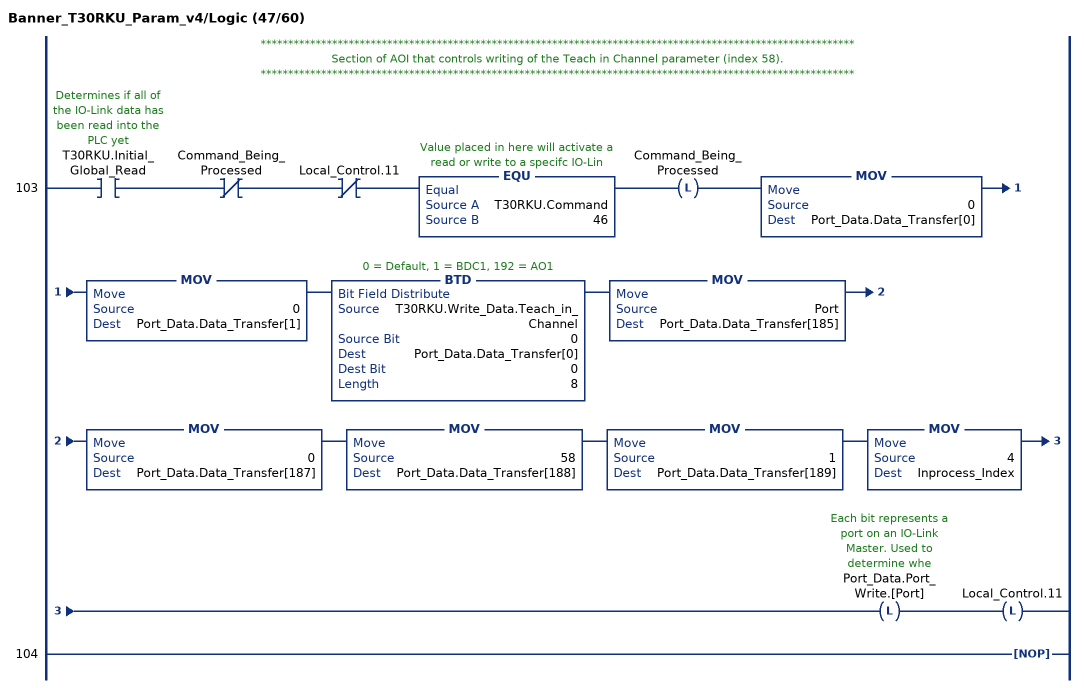
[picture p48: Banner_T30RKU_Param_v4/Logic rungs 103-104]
   // ************************************************************************************************************
   // Section of AOI that controls writing of the Teach in Channel parameter (index 58).
   // ************************************************************************************************************
   103: XIC(T30RKU.Initial_Global_Read)XIO(Command_Being_Processed)XIO(Local_Control.11)EQU(T30RKU.Command,46)OTL(Command_Being_Processed)MOV(0,Port_Data.Data_Transfer[0])MOV(0,Port_Data.Data_Transfer[1])BTD(T30RKU.Write_Data.Teach_in_Channel,0,Port_Data.Data_Transfer[0],0,8)MOV(Port,Port_Data.Data_Transfer[185])MOV(0,Port_Data.Data_Transfer[187])MOV(58,Port_Data.Data_Transfer[188])MOV(1,Port_Data.Data_Transfer[189])MOV(4,Inprocess_Index)OTL(Port_Data.Port_Write.[Port])OTL(Local_Control.11);
   104: NOP();
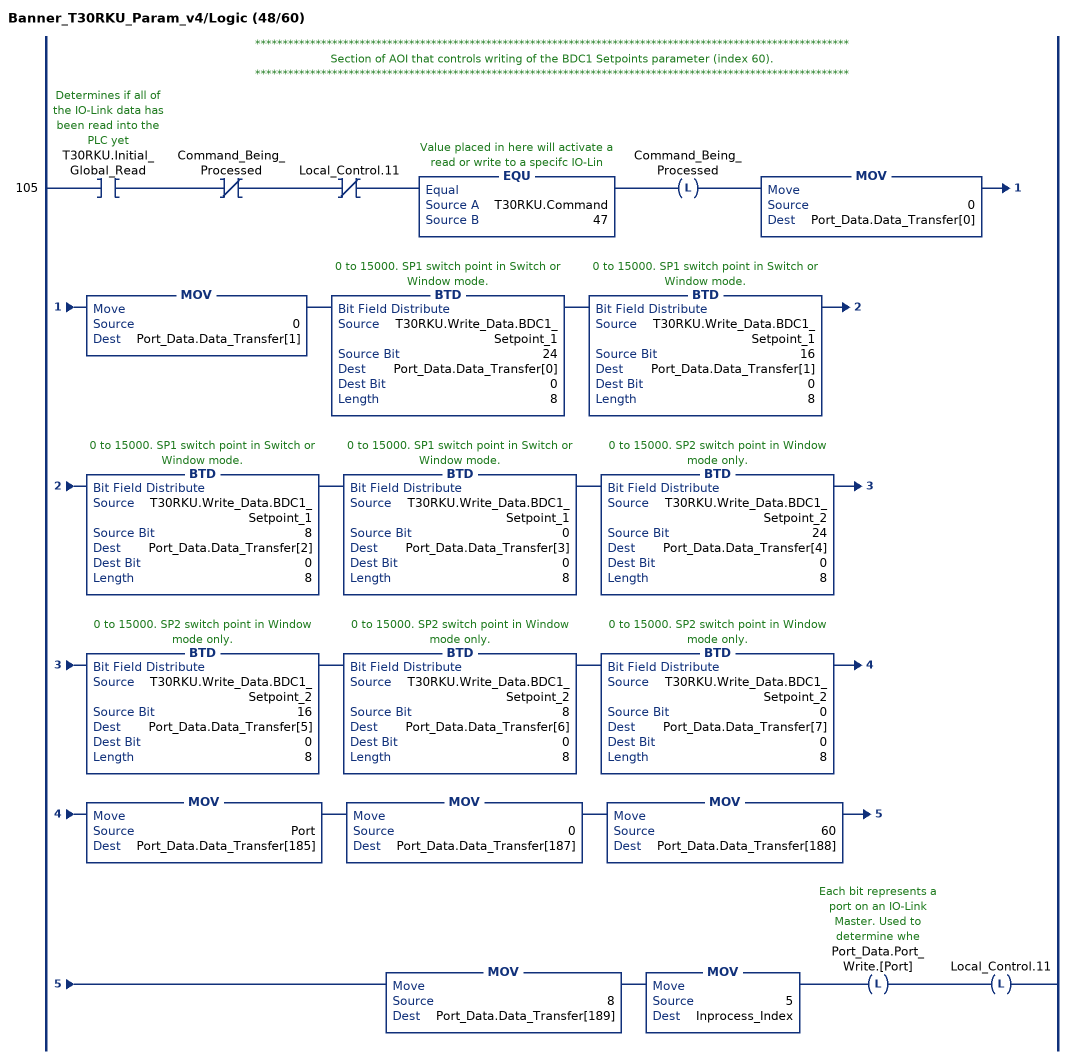
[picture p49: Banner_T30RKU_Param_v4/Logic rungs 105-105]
   // ************************************************************************************************************
   // Section of AOI that controls writing of the BDC1 Setpoints parameter (index 60).
   // ************************************************************************************************************
   105: XIC(T30RKU.Initial_Global_Read)XIO(Command_Being_Processed)XIO(Local_Control.11)EQU(T30RKU.Command,47)OTL(Command_Being_Processed)MOV(0,Port_Data.Data_Transfer[0])MOV(0,Port_Data.Data_Transfer[1])BTD(T30RKU.Write_Data.BDC1_Setpoint_1,24,Port_Data.Data_Transfer[0],0,8)BTD(T30RKU.Write_Data.BDC1_Setpoint_1,16,Port_Data.Data_Transfer[1],0,8)BTD(T30RKU.Write_Data.BDC1_Setpoint_1,8,Port_Data.Data_Transfer[2],0,8)BTD(T30RKU.Write_Data.BDC1_Setpoint_1,0,Port_Data.Data_Transfer[3],0,8)BTD(T30RKU.Write_Data.BDC1_Setpoint_2,24,Port_Data.Data_Transfer[4],0,8)BTD(T30RKU.Write_Data.BDC1_Setpoint_2,16,Port_Data.Data_Transfer[5],0,8)BTD(T30RKU.Write_Data.BDC1_Setpoint_2,8,Port_Data.Data_Transfer[6],0,8)BTD(T30RKU.Write_Data.BDC1_Setpoint_2,0,Port_Data.Data_Transfer[7],0,8)MOV(Port,Port_Data.Data_Transfer[185])MOV(0,Port_Data.Data_Transfer[187])MOV(60,Port_Data.Data_Transfer[188])MOV(8,Port_Data.Data_Transfer[189])MOV(5,Inprocess_Index)OTL(Port_Data.Port_Write.[Port])OTL(Local_Control.11);
